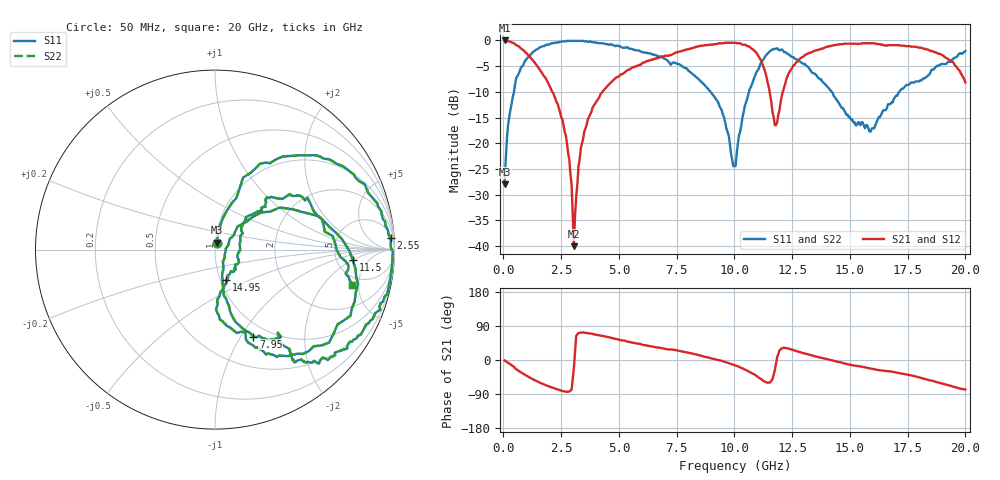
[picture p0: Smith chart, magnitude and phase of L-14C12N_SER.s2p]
#	mhz	s	ma	r	50
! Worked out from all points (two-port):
!   400 points, 50 MHz to 20 GHz, reference 50 ohm
!   highest |S21| = 0.00 dB at 50 MHz (marker M1); lowest = -40.0 dB at 3.05 GHz (marker M2)
!   |S21| within 3 dB of the highest: 6.99 GHz to 11.04 GHz (4.047 GHz wide, 44.9 % of centre); 13.02 GHz to 19.06 GHz (6.035 GHz wide, 37.6 % of centre)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
!   lowest |S11| = -28.0 dB at 50 MHz (marker M3), VSWR 1.08, Z = 50.8 + j3.96 ohm
!   |S11| at or under -10 dB: start of sweep to 455.6 MHz; 8.969 GHz to 10.63 GHz (1.659 GHz wide, 16.9 % of centre); 14.22 GHz to 17.13 GHz (2.913 GHz wide, 18.6 % of centre)
!   |S22| runs from -28.0 to -0.1 dB; largest |S21 - S12| = 0
!   S11 on the Smith chart (normalised r, x): 50 MHz: 1.02, +0.08; 2.55 GHz: 8, +28; 7.95 GHz: 0.84, -1.14; 11.5 GHz: 7.11, -2.02; 14.95 GHz: 1.07, -0.37; 20 GHz: 4.04, -4.19
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50  0.04 76.4  1 -1.3  1 -1.3  0.04 76.4
200  0.15 77.2  0.98 -7.3  0.98 -7.3  0.15 77.2
550  0.43 68.7  0.9 -24.3  0.9 -24.3  0.43 68.7
1300  0.78 41.9  0.63 -51.6  0.63 -51.6  0.78 41.9
2550  0.98 3.8  0.17 -81.9  0.17 -81.9  0.98 3.8
2950  0.99 -5.0  0.04 -78.5  0.04 -78.5  0.99 -5.0
3050  0.99 -7.2  0.01 -21.2  0.01 -21.2  0.99 -7.2
3400  0.99 -13.7  0.1 72.5  0.1 72.5  0.99 -13.7
4400  0.93 -32.2  0.34 62.1  0.34 62.1  0.93 -32.2
6700  0.7 -53.6  0.68 32.8  0.68 32.8  0.7 -53.6
7950  0.53 -66.2  0.82 19.8  0.82 19.8  0.53 -66.2
9300  0.25 -78.8  0.93 0.1  0.93 0.1  0.25 -78.8
10050  0.06 4.0  0.95 -14.4  0.95 -14.4  0.06 4.0
10650  0.33 38.8  0.87 -30.9  0.87 -30.9  0.33 38.8
11500  0.77 -4.3  0.34 -59.6  0.34 -59.6  0.77 -4.3
11800  0.83 -23.3  0.15 -9.9  0.15 -9.9  0.83 -23.3
12350  0.73 -53.3  0.48 30.0  0.48 30.0  0.73 -53.3
13350  0.49 -69.8  0.77 12.0  0.77 12.0  0.49 -69.8
14950  0.18 -69.5  0.93 -11.8  0.93 -11.8  0.18 -69.5
16700  0.24 44.6  0.9 -29.8  0.9 -29.8  0.24 44.6
18950  0.59 29.3  0.73 -61.5  0.73 -61.5  0.59 29.3
20000  0.79 -14.3  0.39 -77.7  0.39 -77.7  0.79 -14.3
